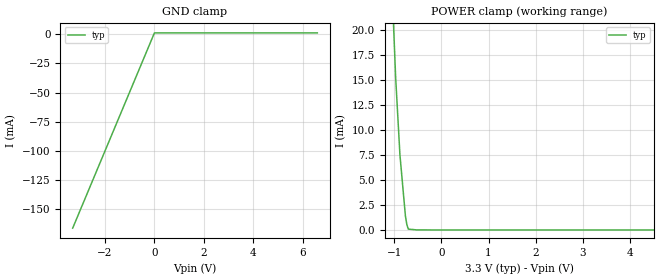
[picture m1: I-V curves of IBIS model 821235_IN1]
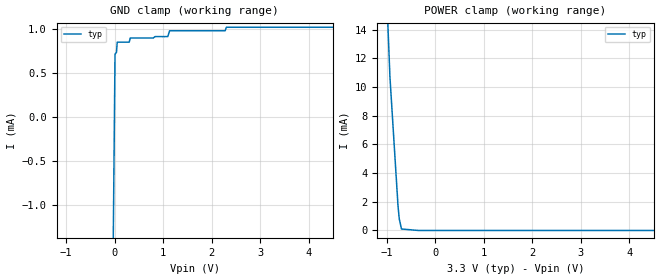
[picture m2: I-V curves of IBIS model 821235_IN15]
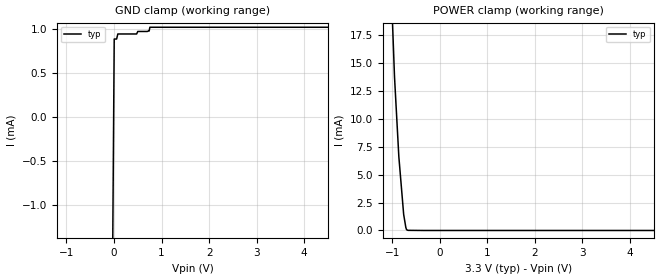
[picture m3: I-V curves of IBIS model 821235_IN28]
| COPYRIGHT(C) MENTOR GRAPHICS CORPORATION 2002 ALL
| RIGHTS RESERVED. THIS WORK CONTAINS PROPRIETARY
| INFORMATION WHICH IS THE PROPERTY OF MENTOR GRAPHICS
| CORPORATION OR ITS LICENSORS. USE OF THESE MATERIALS
| IS SUBJECT TO THE TERMS BELOW.
| USE: MENTOR GRAPHICS HAS LICENSED IBIS MODELS TO
| SPECIFIC INTEGRATED CIRCUIT SUPPLIERS ("IC VENDORS")
| FOR USE AND DISTRIBUTION AS FOLLOWS: EACH IC VENDOR
| MAY USE IBIS MODELS, AND DISTRIBUTE THEM TO IC VENDOR'S
| CUSTOMERS TO USE, SOLELY FOR DEVELOPING PRINTED
| CIRCUIT BOARD DESIGNS. NO OTHER USE OR DISTRIBUTION
| OF THESE MATERIALS IS PERMITTED.
| DISCLAIMER OF WARRANTY:  UNLESS OTHERWISE AGREED
| IN WRITING, MENTOR GRAPHICS SOFTWARE AND ASSOCIATED
| FILES ARE PROVIDED "AS IS" AND WITHOUT WARRANTY.
| MENTOR GRAPHICS HAS NO OBLIGATION TO SUPPORT OR
| OTHERWISE MAINTAIN SOFTWARE.  MENTOR GRAPHICS MAKES
| NO WARRANTIES, EXPRESS OR IMPLIED WITH RESPECT TO
| SOFTWARE INCLUDING ANY WARRANTY OF MERCHANTABILITY
| OR FITNESS FOR A PARTICULAR PURPOSE.
| LIMITATION OF LIABILITY:  MENTOR GRAPHICS IS NOT LIABLE FOR
| ANY PROPERTY DAMAGE, PERSONAL INJURY, LOSS OF PROFITS,
| INTERRUPTION OF BUSINESS, OR FOR ANY OTHER SPECIAL,
| CONSEQUENTIAL OR INCIDENTAL DAMAGES, HOWEVER CAUSED,
| WHETHER FOR BREACH OF WARRANTY, CONTRACT, TORT
| (INCLUDING NEGLIGENCE), STRICT LIABILITY OR OTHERWISE. IN NO
| EVENT SHALL MENTOR GRAPHICS' LIABILITY EXCEED THE AMOUNT
| PAID FOR THE PRODUCT GIVING RISE TO THE CLAIM.
| TRADEMARKS:  THE FOLLOWING ARE REGISTERED TRADEMARKS
| OR SERVICE MARKS OF MENTOR GRAPHICS CORPORATION:
| ICX, ICX STANDARD LIBRARY, ICX PROJECT MODELING,
| AND ICX CUSTOM MODELING.  THE FOLLOWING ARE TRADEMARKS
| OR SERVICE MARKS OF MENTOR GRAPHICS CORPORATION:
| QUALITYIBIS, MODELVIEWER, AND MODELEDITOR. ALL OTHER
| BRANDS AND PRODUCT NAMES ARE TRADEMARKS OF THEIR
| RESPECTIVE OWNERS.
| COPIES:  ALL COPIES OF SOFTWARE, INCLUDING BUT NOT LIMITED
| TO ANY MODIFICATIONS, ENHANCEMENTS OR DERIVATIVE WORKS
| MUST CONTAIN ALL MENTOR GRAPHICS' NOTICES AND LEGENDS,
| INCLUDING THOSE EMBEDDED IN SOFTWARE AND THOSE AFFIXED
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[IBIS Ver] 3.2
[File Name] ad9752ar_3v.ibs
[File Rev] 2.0
[Source] Measured and created by ICX Technology
[Date] Friday 7/5/02 11:58:39 AM
[Copyright]
| COPYRIGHT(C) MENTOR GRAPHICS CORPORATION 2002 ALL
| RIGHTS RESERVED. THIS WORK CONTAINS PROPRIETARY
| INFORMATION WHICH IS THE PROPERTY OF MENTOR GRAPHICS
| CORPORATION OR ITS LICENSORS. USE OF THESE MATERIALS
| IS SUBJECT TO THE TERMS BELOW.
| USE: MENTOR GRAPHICS HAS LICENSED IBIS MODELS TO
| SPECIFIC INTEGRATED CIRCUIT SUPPLIERS ("IC VENDORS")
| FOR USE AND DISTRIBUTION AS FOLLOWS: EACH IC VENDOR
| MAY USE IBIS MODELS, AND DISTRIBUTE THEM TO IC VENDOR'S
| CUSTOMERS TO USE, SOLELY FOR DEVELOPING PRINTED
| CIRCUIT BOARD DESIGNS. NO OTHER USE OR DISTRIBUTION
| OF THESE MATERIALS IS PERMITTED.
|  ZAP Model Builder 3.2
[Component] AD9752AR_3v
[Manufacturer] AnalogDevices
[Package]
| variable   typ   min   max
R_pkg  .182ohms NA NA
L_pkg  4.914nH NA NA
C_pkg  .654pF NA NA
[Pin] signal_name  model_name  R_pin  L_pin C_pin
1 DB11 821235_IN1 .194 6.364n .744p
2 DB10 821235_IN4 .19 5.864n .714p
3 DB9 821235_IN4 .186 5.374n .684p
4 DB8 821235_IN4 .182 4.894n .654p
5 DB7 821235_IN4 .178 4.424n .624p
6 DB6 821235_IN4 .174 3.964n .594p
7 DB5 821235_IN9 .17 3.514n .564p
8 DB4 821235_IN9 .17 3.514n .564p
9 DB3 821235_IN9 .174 3.964n .594p
10 DB2 821235_IN9 .178 4.424n .624p
11 DB1 821235_IN9 .182 4.894n .654p
12 DB0 821235_IN1 .186 5.374n .684p
13 NC NC .19 5.864n .714p
14 NC NC .194 6.364n .744p
15 SLEEP 821235_IN15 .194 6.364n .744p
16 REFLO NC .19 5.864n .714p
17 REFIO NC .186 5.374n .684p
18 FSADJ NC .182 4.894n .654p
19 NC NC .178 4.424n .624p
20 ACOM GND .174 3.964n .594p
21 IOUTB NC .17 3.514n .564p
22 IOUTA NC .17 3.514n .564p
23 ICOMP NC .174 3.964n .594p
24 AVDD POWER .178 4.424n .624p
25 NC NC .182 4.894n .654p
26 DCOM GND .186 5.374n .684p
27 DVDD POWER .19 5.864n .714p
28 CLOCK 821235_IN28 .194 6.364n .744p
| Models and submodels in the file (5): 821235_IN1 (Input), 821235_IN15 (Input), 821235_IN28 (Input), 821235_IN4 (Input), 821235_IN9 (Input)
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| COPYRIGHT(C) MENTOR GRAPHICS CORPORATION 2002 ALL
| RIGHTS RESERVED. THIS WORK CONTAINS PROPRIETARY
| INFORMATION WHICH IS THE PROPERTY OF MENTOR GRAPHICS
| CORPORATION OR ITS LICENSORS. USE OF THESE MATERIALS
| IS SUBJECT TO THE TERMS BELOW.
| USE: MENTOR GRAPHICS HAS LICENSED IBIS MODELS TO
| SPECIFIC INTEGRATED CIRCUIT SUPPLIERS ("IC VENDORS")
| FOR USE AND DISTRIBUTION AS FOLLOWS: EACH IC VENDOR
| MAY USE IBIS MODELS, AND DISTRIBUTE THEM TO IC VENDOR'S
| CUSTOMERS TO USE, SOLELY FOR DEVELOPING PRINTED
| CIRCUIT BOARD DESIGNS. NO OTHER USE OR DISTRIBUTION
| OF THESE MATERIALS IS PERMITTED.
| Model Application Version 1.89 2/18/99.
[Model] 821235_IN1
Model_type Input
Vinl = 900.0mV
Vinh = 2.100V
C_comp 5.000pF NA NA
| variable typ   min   max
[Voltage Range] 3.300V NA NA
[GND Clamp Reference] 0.000V NA NA
[POWER Clamp Reference] 3.300V NA NA
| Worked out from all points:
|   POWER clamp passes 1 mA (typ) near -0.75 V on its own axis
[GND Clamp]
-3.3V     -166mA     NA         NA
5.284mV   1.005mA    NA         NA
20.36mV   1.14mA     NA         NA
6.6V      1.14mA     NA         NA
[POWER Clamp]
-3.3V     391.2mA    NA         NA
-1.058V   25.95mA    NA         NA
-967.2mV  15.3mA     NA         NA
-876.1mV  7.513mA    NA         NA
-759.5mV  1.384mA    NA         NA
-729mV    525.5uA    NA         NA
-698.5mV  88.65uA    NA         NA
-683.6mV  80.97uA    NA         NA
-526.3mV  8.45uA     NA         NA
-369.1mV  8.45uA     NA         NA
-184.6mV  0A         NA         NA
6.6V      0A         NA         NA
| COPYRIGHT(C) MENTOR GRAPHICS CORPORATION 2002 ALL
| RIGHTS RESERVED. THIS WORK CONTAINS PROPRIETARY
| INFORMATION WHICH IS THE PROPERTY OF MENTOR GRAPHICS
| CORPORATION OR ITS LICENSORS. USE OF THESE MATERIALS
| IS SUBJECT TO THE TERMS BELOW.
| USE: MENTOR GRAPHICS HAS LICENSED IBIS MODELS TO
| SPECIFIC INTEGRATED CIRCUIT SUPPLIERS ("IC VENDORS")
| FOR USE AND DISTRIBUTION AS FOLLOWS: EACH IC VENDOR
| MAY USE IBIS MODELS, AND DISTRIBUTE THEM TO IC VENDOR'S
| CUSTOMERS TO USE, SOLELY FOR DEVELOPING PRINTED
| CIRCUIT BOARD DESIGNS. NO OTHER USE OR DISTRIBUTION
| OF THESE MATERIALS IS PERMITTED.
| Model Application Version 1.89 2/18/99.
[Model] 821235_IN15
Model_type Input
Vinl = 900.0mV
Vinh = 2.100V
C_comp 5.000pF NA NA
| variable typ   min   max
[Voltage Range] 3.300V NA NA
[GND Clamp Reference] 0.000V NA NA
[POWER Clamp Reference] 3.300V NA NA
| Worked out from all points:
|   POWER clamp passes 1 mA (typ) near -0.75 V on its own axis
[GND Clamp]
-3.3V     -191.8mA   NA         NA
5.326mV   710.2uA    NA         NA
35.59mV   733.3uA    NA         NA
50.87mV   847.3uA    NA         NA
297.1mV   847.3uA    NA         NA
319.4mV   893.9uA    NA         NA
791.8mV   893.9uA    NA         NA
1.093V    910.3uA    NA         NA
1.13V     976.4uA    NA         NA
2.275V    976.4uA    NA         NA
2.301V    1.016mA    NA         NA
6.6V      1.016mA    NA         NA
[POWER Clamp]
-3.3V     260.4mA    NA         NA
-1.089V   23.78mA    NA         NA
-936.7mV  10.72mA    NA         NA
-769.5mV  1.69mA     NA         NA
-744.1mV  808.7uA    NA         NA
-698.4mV  102uA      NA         NA
-349.2mV  0A         NA         NA
6.6V      0A         NA         NA
| COPYRIGHT(C) MENTOR GRAPHICS CORPORATION 2002 ALL
| RIGHTS RESERVED. THIS WORK CONTAINS PROPRIETARY
| INFORMATION WHICH IS THE PROPERTY OF MENTOR GRAPHICS
| CORPORATION OR ITS LICENSORS. USE OF THESE MATERIALS
| IS SUBJECT TO THE TERMS BELOW.
| USE: MENTOR GRAPHICS HAS LICENSED IBIS MODELS TO
| SPECIFIC INTEGRATED CIRCUIT SUPPLIERS ("IC VENDORS")
| FOR USE AND DISTRIBUTION AS FOLLOWS: EACH IC VENDOR
| MAY USE IBIS MODELS, AND DISTRIBUTE THEM TO IC VENDOR'S
| CUSTOMERS TO USE, SOLELY FOR DEVELOPING PRINTED
| CIRCUIT BOARD DESIGNS. NO OTHER USE OR DISTRIBUTION
| OF THESE MATERIALS IS PERMITTED.
| Model Application Version 1.89 2/18/99.
[Model] 821235_IN28
Model_type Input
Vinl = 900.0mV
Vinh = 2.100V
C_comp 5.000pF NA NA
| variable typ   min   max
[Voltage Range] 3.300V NA NA
[GND Clamp Reference] 0.000V NA NA
[POWER Clamp Reference] 3.300V NA NA
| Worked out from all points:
|   POWER clamp passes 1 mA (typ) near -0.74 V on its own axis
[GND Clamp]
-3.3V     -246.5mA   NA         NA
5.286mV   886.3uA    NA         NA
55.96mV   886.3uA    NA         NA
81.3mV    943.7uA    NA         NA
476.8mV   943.7uA    NA         NA
501.5mV   972.1uA    NA         NA
700.1mV   972.1uA    NA         NA
724.9mV   977.5uA    NA         NA
740.1mV   977.5uA    NA         NA
755.3mV   1.02mA     NA         NA
6.6V      1.02mA     NA         NA
[POWER Clamp]
-3.3V     400.6mA    NA         NA
-1.043V   24.22mA    NA         NA
-952.1mV  13.77mA    NA         NA
-860.8mV  6.606mA    NA         NA
-759.4mV  1.435mA    NA         NA
-713.8mV  270.1uA    NA         NA
-698.4mV  73.69uA    NA         NA
-668.3mV  12.28uA    NA         NA
-334.1mV  0A         NA         NA
6.6V      0A         NA         NA
